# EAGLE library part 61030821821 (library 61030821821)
WURTH ELEKTRONIK - 61030821821 - PCB Receptacle, Board-to-Board, 2.54 mm, 2 Rows, 8 Contacts, Surface Mount, WR-PHD Series Source: Datasheet
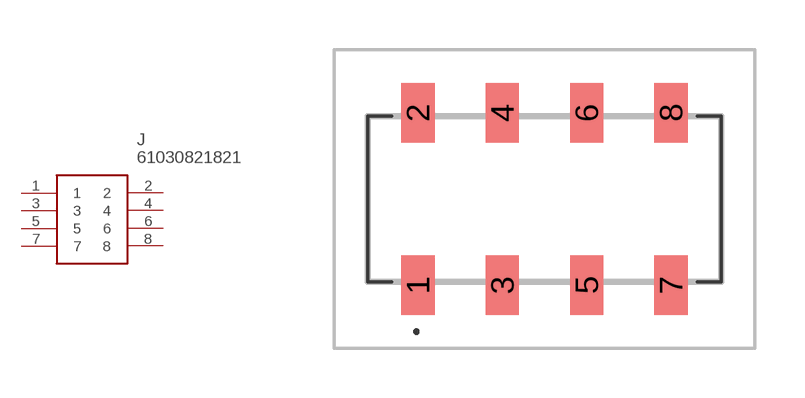
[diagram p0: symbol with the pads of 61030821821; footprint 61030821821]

Designator prefix J

## 61030821821 (Description: WURTH ELEKTRONIK - 61030821821 - PCB Receptacle, Board-to-Board, 2.54 mm, 2 Rows, 8 Contacts, Surface Mount, WR-PHD Series; Height: 7.75mm; Manufacturer_Name: Wurth Elektronik; Manufacturer_Part_Number: 61030821821; Mouser_Part_Number: 710-61030821821; Mouser_Price-Stock: https://www.mouser.co.uk/ProductDetail/Wurth-Elektronik/61030821821?qs=Cb2nCFKsA8oJEHHhLPQ3%2Fg%3D%3D)  [61030821821]
1  1
2  2
3  3
4  4
5  5
6  6
7  7
8  8

## Footprint 61030821821 (pad centres in mm)
61030821821-2
smd 1 x 1.8: 1 -3.81,-2.6; 2 -3.81,2.6; 3 -1.27,-2.6; 4 -1.27,2.6; 5 1.27,-2.6; 6 1.27,2.6; 7 3.81,-2.6; 8 3.81,2.6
